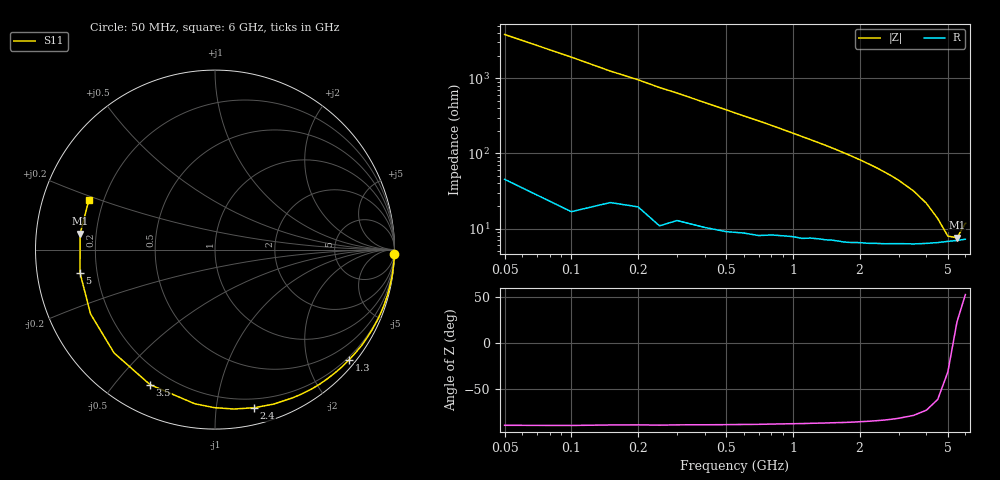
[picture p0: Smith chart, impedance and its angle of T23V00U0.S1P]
! SIEMENS Discrete & RF Semiconductors
! BAS70-04W
! Si Schottky Diode in SOT323
! VR = 3 V
! S-Parameters:  November  1997
# GHz  S  MA  R  50
!  f  S11
! GHz  MAG  ANG
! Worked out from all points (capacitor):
!   34 points, 50 MHz to 6 GHz, reference 50 ohm
!   read as one part to ground: C = 833 fF near 50 MHz
!   lowest |Z| = 7.54 ohm at 5.5 GHz (marker M1)
!   series resonance near 5.294 GHz, so ESL is about 1.1 nH
!   S11 on the Smith chart (normalised r, x): 50 MHz: 1, -76; 1.3 GHz: 0.15, -2.79; 2.4 GHz: 0.13, -1.27; 3.5 GHz: 0.13, -0.62; 5 GHz: 0.14, -0.08; 6 GHz: 0.14, +0.19
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0.05  0.9997 -1.5
0.25  0.9981 -7.6
0.4  0.9955 -12.0
0.5  0.9938 -15.0
0.6  0.9915 -18.0
0.7  0.9894 -20.9
0.8  0.986 -23.9
0.9  0.9827 -27.0
1.1  0.9761 -33.2
1.3  0.9672 -39.4
1.4  0.9633 -42.5
1.5  0.9584 -45.7
1.6  0.9539 -49.0
1.7  0.9496 -52.3
1.8  0.9445 -55.6
1.9  0.9383 -59.0
2  0.9323 -62.4
2.2  0.9208 -69.2
2.4  0.9076 -76.1
2.6  0.8944 -83.3
2.8  0.8804 -90.3
3  0.8662 -97.5
3.5  0.835 -115.7
4  0.8048 -134.3
4.5  0.7805 -152.7
5  0.7633 -170.3
5.5  0.7564 173.2
6  0.7552 158.5
